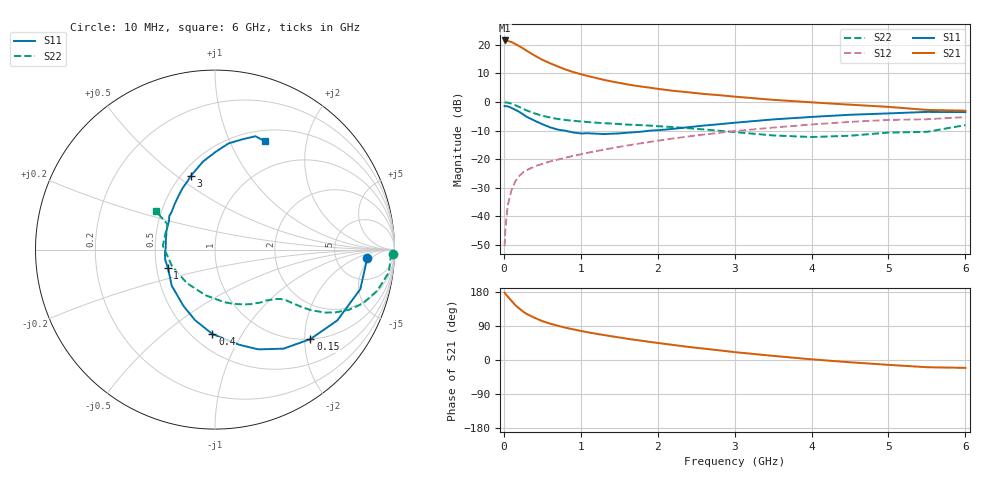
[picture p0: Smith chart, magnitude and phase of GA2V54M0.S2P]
! Infineon Technologies  Discrete & RF Semiconductors
! BF775
! Si NPN RF Bipolar Junction Transistor in SOT23
! VCE = 2.5 V  IC = 4 mA
! Common Emitter S-Parameters:  May  1996
# GHz  S  MA  R  50
!  f  S11  S21  S12  S22
! GHz  MAG  ANG  MAG  ANG  MAG  ANG  MAG  ANG
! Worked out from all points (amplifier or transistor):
!   36 points, 10 MHz to 6 GHz, reference 50 ohm
!   highest |S21| = 21.5 dB at 10 MHz (marker M1)
!   |S21| within 3 dB of that: start of sweep to 262.6 MHz
!   unconditionally stable (mu >= 1): 857 MHz to 3.814 GHz
!   at 250 MHz: K = 0.43, MSG = 21.7 dB, |S12| = -24.6 dB
!   at 1.4 GHz: K = 1.14, MAG = 9.4 dB, |S12| = -16.2 dB
!   at 6 GHz: K = 0.99, MSG = 1.1 dB, |S12| = -5.3 dB
!   S11 on the Smith chart (normalised r, x): 10 MHz: 11, -4; 150 MHz: 1.00, -2.13; 400 MHz: 0.62, -0.75; 1 GHz: 0.57, -0.13; 3 GHz: 0.56, +0.57; 6 GHz: 0.63, +1.37
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0.01  0.8485 -3.2  11.92 177.6  0.003 87.1  0.9932 -1.4
0.02  0.8433 -6.3  11.86 174.8  0.0061 91.0  0.9792 -3.0
0.05  0.839 -15.2  11.69 167.6  0.0153 82.0  0.9767 -7.5
0.1  0.7874 -30.1  11.2 156.0  0.029 74.0  0.9328 -14.2
0.15  0.7286 -43.2  10.33 144.7  0.041 67.3  0.8759 -20.1
0.2  0.6712 -55.3  9.488 135.9  0.0508 63.2  0.818 -24.2
0.25  0.6062 -66.5  8.656 127.7  0.0586 59.2  0.7589 -27.4
0.3  0.5479 -75.6  7.835 121.2  0.0645 57.1  0.7083 -29.7
0.4  0.471 -91.7  6.498 111.4  0.0746 53.7  0.6313 -32.3
0.5  0.4086 -105.8  5.475 102.7  0.0827 52.3  0.5751 -33.6
0.6  0.3605 -119.0  4.764 96.1  0.091 52.1  0.5344 -34.4
0.7  0.3288 -130.2  4.194 90.4  0.0979 52.4  0.5053 -35.1
0.8  0.3139 -140.3  3.71 85.4  0.1057 52.6  0.4837 -35.5
1  0.2817 -159.0  3.063 76.7  0.1214 53.0  0.4561 -37.1
1.1  0.2832 -168.8  2.831 72.9  0.1298 53.4  0.4447 -38.3
1.6  0.2896 159.0  2.034 56.2  0.1729 53.3  0.4027 -44.7
2.2  0.3386 131.7  1.57 39.8  0.2296 50.2  0.3638 -56.6
3  0.4331 108.0  1.241 20.8  0.3091 43.0  0.2974 -80.0
3.5  0.4954 97.7  1.091 10.9  0.3567 37.2  0.2598 -101.9
4.5  0.5972 82.6  0.897 -6.0  0.4482 24.3  0.2567 -159.3
5.5  0.6705 70.4  0.726 -19.0  0.4989 9.3  0.3004 151.9
6  0.6646 65.1  0.703 -20.8  0.5429 5.2  0.3937 146.9
